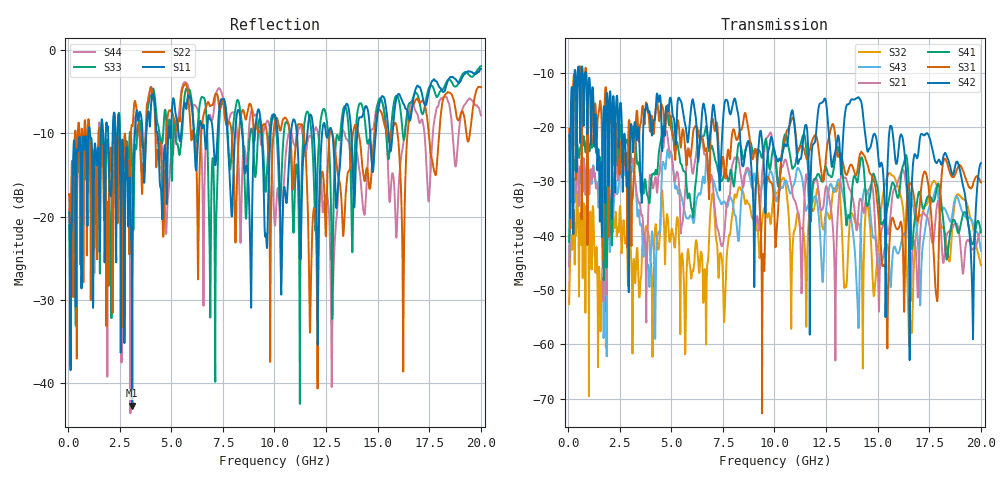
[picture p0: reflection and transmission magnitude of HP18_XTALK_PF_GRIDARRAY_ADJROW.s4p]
# MHz S MA R 50.00
! FREQ  S11  S12  S13  S14
!  S21  S22  S23  S24
!  S31  S32  S33  S34
!  S41  S42  S43  S44
!  MAG  ANG  MAG  ANG  MAG  ANG  MAG  ANG
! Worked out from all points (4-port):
!   1996 points, 50 MHz to 20 GHz, reference 50 ohm
!   strongest paths, dB at 50 MHz, 5.04 GHz, 10.03 GHz, 15.02 GHz, 20 GHz:
!     S42: -21.5, -16.8, -25.1, -25.0, -26.6
!     S31: -20.3, -21.1, -40.5, -35.5, -30.2
!     S41: -41.1, -20.0, -24.9, -31.7, -39.4
!     S21: -45.7, -25.8, -26.5, -47.5, -38.8
!     S43: -45.3, -26.0, -32.2, -45.2, -42.8
!     S32: -52.6, -38.9, -32.3, -41.9, -45.4
!   lowest |S11| = -42.7 dB at 3.11 GHz (marker M1), VSWR 1.01, Z = 49.5 - j0.517 ohm
!   |S11| at or under -10 dB: start of sweep to 990.4 MHz; 2.496 GHz to 3.241 GHz (745.6 MHz wide, 26 % of centre); 10.15 GHz to 10.8 GHz (648.3 MHz wide, 6.19 % of centre)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
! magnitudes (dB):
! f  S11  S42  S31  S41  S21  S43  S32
! 50 MHz  -19.5  -21.5  -20.3  -41.1  -45.7  -45.3  -52.6
! 3.11 GHz  -42.7  -22.2  -33.2  -20.2  -26.4  -27.3  -54.2
! 14.07 GHz  -8.5  -14.5  -26.6  -29.0  -35.1  -57.0  -37.7
! 15.44 GHz  -7.6  -32.1  -53.6  -35.4  -38.6  -41.5  -29.4
! 16.59 GHz  -8.3  -39.0  -30.4  -37.9  -51.6  -32.2  -56.2
! 19.59 GHz  -2.7  -52.2  -30.9  -41.5  -42.6  -37.3  -37.8
! 20 GHz  -2.3  -26.6  -30.2  -39.4  -38.8  -42.8  -45.4
